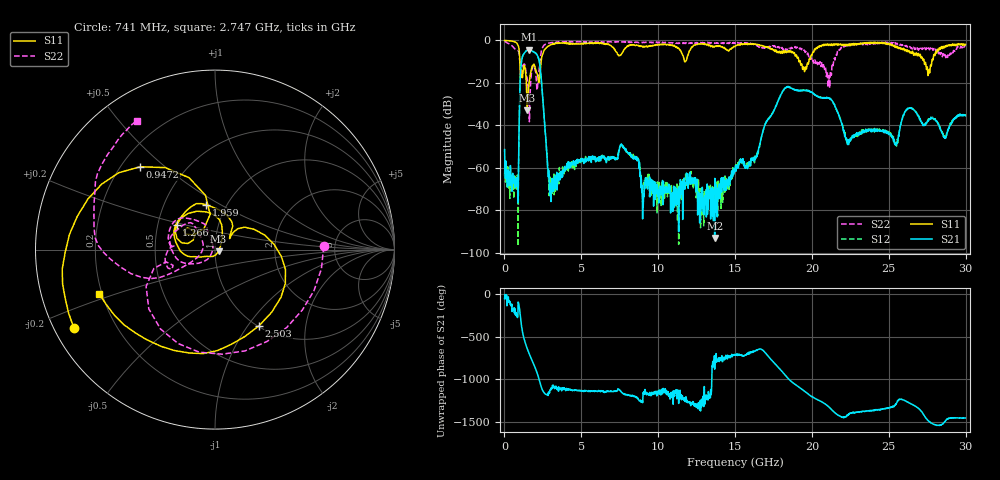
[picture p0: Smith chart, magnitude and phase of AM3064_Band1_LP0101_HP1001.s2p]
# Hz S DB R 50.0
!freq dBS11 angS11 dBS21 angS21 dBS12 angS12 dBS22 angS22
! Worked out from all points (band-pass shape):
!   1600 points, 10 MHz to 29.98 GHz, reference 50 ohm
!   highest |S21| = -4.43 dB at 1.584 GHz (marker M1); lowest = -93.1 dB at 13.67 GHz (marker M2)
!   |S21| within 3 dB of the highest: 1.182 GHz to 2.165 GHz (983.5 MHz wide, 58.8 % of centre)
!   lowest |S11| = -33.0 dB at 1.472 GHz (marker M3), VSWR 1.05, Z = 52 - j1.01 ohm
!   |S11| at or under -10 dB: 1.002 GHz to 2.385 GHz (1.383 GHz wide, 81.7 % of centre); 19.24 GHz to 19.79 GHz (554.4 MHz wide, 2.84 % of centre); 27.3 GHz to 27.8 GHz (495.2 MHz wide, 1.8 % of centre)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
!   |S22| runs from -38.3 to -0.4 dB; largest |S21 - S12| = 0.0072
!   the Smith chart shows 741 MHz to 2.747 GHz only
!   S11 on the Smith chart (normalised r, x): 741 MHz: 0.06, -0.26; 947.2 MHz: 0.28, +0.42; 1.266 GHz: 0.63, +0.19; 1.959 GHz: 0.80, +0.43; 2.503 GHz: 1.02, -1.13; 2.747 GHz: 0.19, -0.18
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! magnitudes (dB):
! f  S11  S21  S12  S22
! 10 MHz  0.0  -51.4  -64.0  -0.4
! 741 MHz  -0.9  -65.1  -67.7  -4.4
! 947.2 MHz  -4.1  -43.7  -43.3  -6.1
! 1.266 GHz  -11.9  -6.3  -6.2  -11.2
! 1.472 GHz  -33.0  -4.7  -4.6  -17.8
! 1.584 GHz  -21.1  -4.4  -4.5  -27.9
! 1.959 GHz  -11.9  -5.7  -5.6  -13.0
! 2.503 GHz  -6.2  -28.2  -28.1  -3.1
! 2.747 GHz  -3.2  -51.8  -53.2  -1.5
! 3.065 GHz  -1.9  -68.6  -66.9  -1.0
! 5.015 GHz  -1.4  -57.2  -56.8  -0.7
! 7.657 GHz  -5.8  -49.7  -49.2  -0.7
! 10 GHz  -2.0  -73.7  -69.6  -0.9
! 13.67 GHz  -2.9  -93.1  -72.4  -1.3
! 15 GHz  -2.7  -60.6  -60.1  -1.4
! 18.23 GHz  -5.6  -22.6  -22.5  -4.3
! 19.99 GHz  -7.1  -24.4  -24.4  -9.2
! 21.12 GHz  -1.8  -27.3  -27.1  -17.4
! 22.33 GHz  -1.8  -47.2  -47.3  -2.5
! 25 GHz  -1.4  -43.6  -42.9  -1.2
! 27.58 GHz  -14.7  -37.6  -36.9  -3.5
! 29.98 GHz  -1.8  -35.6  -35.5  -2.8
